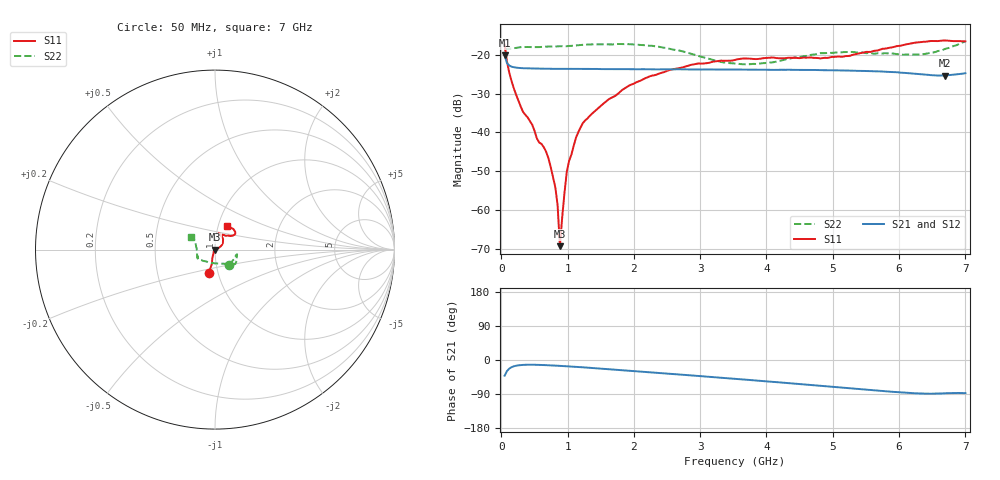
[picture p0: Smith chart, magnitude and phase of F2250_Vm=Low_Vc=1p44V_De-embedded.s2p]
! Integrated Device Technology
! Corporate Headquarters
! 6024 Silver Creek Valley Road
! San Jose, CA 95138  USA
! Phone:  1-408-284-8200
! Toll Free:  1-800-223-1366
! Webpage:  http://www.idt.com/
! Timing and RF Division
! 515 Groton Road, Suite 102
! Westford, MA 01886-6024
! Device:  F2250
! Description: Voltage Variable RF Attenuator
! Frequency:  50.0 -  6000.00 MHz
! Package:  3x3 mm Thin QFN Plastic Package: 16 pin
! Ports:  2 RF, 3 DC
!  Pin  1  = GND
!  Pin  2  = NC
!  Pin  3  = RF1  = Port 1
!  Pin  4  = NC
!  Pin  5  = GND
!  Pin  6  = GND
!  Pin  7  = GND
!  Pin  8  = GND
!  Pin  9  = NC
!  Pin 10  = RF2  = Port 2
!  Pin 11  = NC
!  Pin 12  = GND
!  Pin 13  = GND
!  Pin 14  = VCNTRL
!  Pin 15  = VDD
!  Pin 16  = VMODE
! Vcntrl:  1.440 Volts
! Vmode:  +0.000 Volts
! Vdd:  +3.30  Volts
! Current:  1.192 mA
! Data:  The device was measured on a the F2250 evaluation board which has
!  individual transmission lines to the RF pins.  Data was collected
!  using a calibrated network analyzer.  The evaluation board was
!  de-embedded using a TRL calibration technique.
!  The reference plane is the edge of the package pin.
! Misc:  SN 10
!  Action Tracker AT0258
! Date Measured:  2014-11-26
! Date:  2015-10-15  MJV
! Note:
!  Integrated Device Technology supplies this data as a sample of measured
!  data at the package pin for this product.  Your particular data for this
!  product may vary.
!  Data was taken at 25 degrees C.
!  Integrated Device Technology reserves the right to change this data at anytime.
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# GHz S dB R 50
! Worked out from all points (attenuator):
!   201 points, 50 MHz to 7 GHz, reference 50 ohm
!   highest |S21| = -20.14 dB at 50 MHz (marker M1); lowest = -25.3 dB at 6.687 GHz (marker M2)
!   lowest |S11| = -69.4 dB at 884 MHz (marker M3), VSWR 1.00, Z = 50 - j0.034 ohm
!   |S11| at or under -10 dB: start of sweep to end of sweep
!   |S22| runs from -22.4 to -16.5 dB; largest |S21 - S12| = 0.00029
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0.05  -17.32 -105.2  -20.14 -41.4  -20.13 -41.4  -18.88 -47.3
0.1195  -24.53 -105.0  -22.74 -22.8  -22.73 -22.8  -18.41 -17.9
0.22375  -30.28 -109.9  -23.28 -15.1  -23.28 -15.1  -18.19 -13.3
0.328  -34.70 -115.3  -23.44 -12.9  -23.43 -12.9  -17.98 -12.3
0.467  -38.04 -124.4  -23.49 -12.5  -23.49 -12.5  -18.00 -13.2
0.5365  -41.55 -125.8  -23.55 -12.7  -23.52 -12.7  -17.99 -14.7
0.71025  -46.62 -126.5  -23.57 -13.9  -23.58 -13.9  -17.84 -18.1
0.8145  -54.13 -154.8  -23.60 -14.8  -23.59 -14.8  -17.82 -20.3
0.84925  -58.77 -147.0  -23.59 -15.1  -23.59 -15.1  -17.78 -21.1
0.884  -69.36 -86.9  -23.59 -15.5  -23.58 -15.5  -17.77 -21.9
0.91875  -61.87 17.8  -23.60 -15.8  -23.59 -15.8  -17.75 -22.7
0.98825  -50.12 -18.5  -23.60 -16.5  -23.59 -16.5  -17.75 -23.7
1.12725  -41.33 8.7  -23.61 -18.0  -23.60 -18.0  -17.55 -25.7
1.2315  -37.56 14.0  -23.61 -19.3  -23.61 -19.3  -17.38 -27.7
1.857  -28.67 30.0  -23.67 -27.3  -23.66 -27.3  -17.20 -34.9
2.37825  -24.83 40.4  -23.73 -34.1  -23.71 -34.1  -17.90 -40.8
3.525  -21.29 69.3  -23.80 -49.7  -23.82 -49.7  -22.21 -86.5
4.7065  -20.75 70.7  -23.89 -66.6  -23.90 -66.6  -19.92 -144.7
5.85325  -18.16 38.7  -24.39 -83.3  -24.38 -83.4  -19.65 -163.3
6.33975  -16.68 39.8  -24.99 -88.5  -24.98 -88.6  -19.86 177.8
6.68725  -16.27 47.9  -25.33 -87.8  -25.33 -87.8  -18.50 158.5
7  -16.48 62.7  -24.73 -87.4  -24.74 -87.4  -16.47 151.5
